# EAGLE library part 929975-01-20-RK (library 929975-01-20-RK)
Conn Socket Strip SKT 40 POS 2.54mm Solder ST Thru-Hole Source: Datasheet
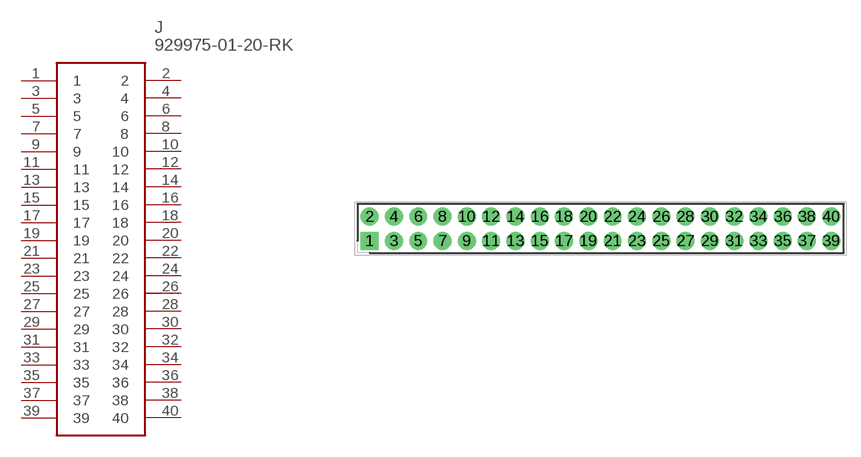
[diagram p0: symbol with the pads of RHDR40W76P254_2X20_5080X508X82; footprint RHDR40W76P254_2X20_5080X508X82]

Designator prefix J

## 929975-01-20-RK (Description: Conn Socket Strip SKT 40 POS 2.54mm Solder ST Thru-Hole; Height: 8.26mm; Manufacturer_Name: 3M; Manufacturer_Part_Number: 929975-01-20-RK; Mouser_Part_Number: 517-929975-01-20-RK; Mouser_Price-Stock: https://www.mouser.co.uk/ProductDetail/3M-Electronic-Solutions-Division/929975-01-20-RK?qs=4V84emjyG36rTUkvYfpt0A%3D%3D)  [RHDR40W76P254_2X20_5080X508X82]
1  1
2  2
3  3
4  4
5  5
6  6
7  7
8  8
9  9
10  10
11  11
12  12
13  13
14  14
15  15
16  16
17  17
18  18
19  19
20  20
21  21
22  22
23  23
24  24
25  25
26  26
27  27
28  28
29  29
30  30
31  31
32  32
33  33
34  34
35  35
36  36
37  37
38  38
39  39
40  40

## Footprint RHDR40W76P254_2X20_5080X508X82 (pad centres in mm)
29975-01-20-RK
drill 1.25 pad 1.875 square: 1 0,0
drill 1.25 pad 1.875: 2 0,2.54; 3 2.54,0; 4 2.54,2.54; 5 5.08,0; 6 5.08,2.54; 7 7.62,0; 8 7.62,2.54; 9 10.16,0; 10 10.16,2.54; 11 12.7,0; 12 12.7,2.54; 13 15.24,0; 14 15.24,2.54; 15 17.78,0; 16 17.78,2.54; 17 20.32,0; 18 20.32,2.54; 19 22.86,0; 20 22.86,2.54; 21 25.4,0; 22 25.4,2.54; 23 27.94,0; 24 27.94,2.54; 25 30.48,0; 26 30.48,2.54; 27 33.02,0; 28 33.02,2.54; 29 35.56,0; 30 35.56,2.54; 31 38.1,0; 32 38.1,2.54; 33 40.64,0; 34 40.64,2.54; 35 43.18,0; 36 43.18,2.54; 37 45.72,0; 38 45.72,2.54; 39 48.26,0; 40 48.26,2.54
